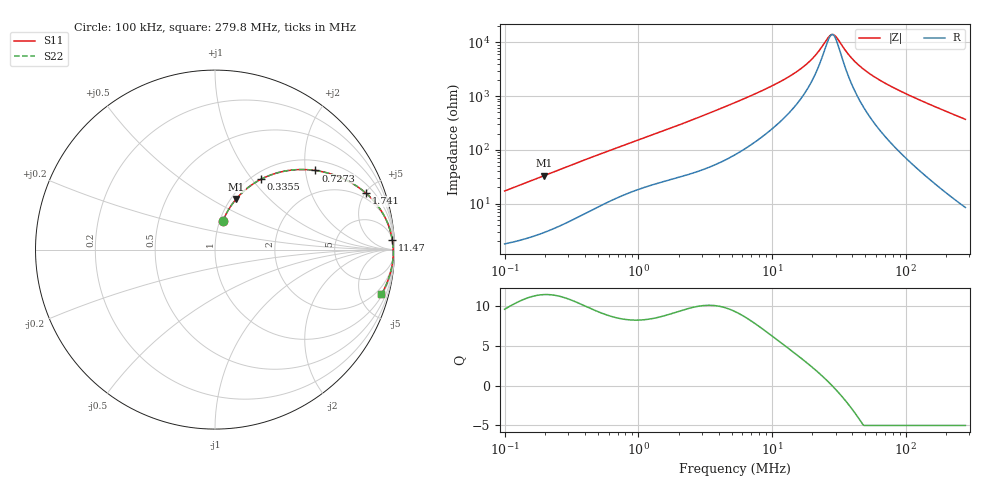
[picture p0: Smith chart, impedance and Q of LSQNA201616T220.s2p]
! LSQNA201616T220  S-PARAMETER MODEL  ( General Type )
! Model Generated by TAIYO YUDEN Corporation (http://www.ty-top.com)
! Version 2.0
! TAIYO YUDEN Control No. 100810NF25SB-FKC
! Copyright(c) 2007 TAIYO YUDEN CO.,LTD. All Rights Reserved.
! Product Description (link to TY-COMPAS)
! https://ds.yuden.co.jp/TYCOMPAS/or/detail?pn=LSQNA201616T220K&u=M
! Products Name : Inductors
! Characteristics :
!  Inductance : 22 uH , SRF(min) : 16 MHz , DC Resistance(max) : 1.3 Ohm
!  Rated Current : Saturation :165 mA , Temp Rise : 370 mA (40 degC)
!  Case Size : 2.0 x 1.6 / 0.079 x 0.063 [mm/inch] , Thickness : 1.6 / 0.063 [mm/inch]
!  (Conditions: Temperature = 25 degC , DC Bias Current/Voltage = 0A / 0V)
! External Node Assignments :
!  1  o---GGG---o  2
! GND o---------o GND
! Frequency Range : 0.1MHz  -  279.750408MHz  [ 402 STEP ]
# MHz S RI R 50
! Freq[MHz].  S11 Real  S11 Imag  S21 Real  S21 Imag  S12 Real  S12 Imag  S22 Real  S22 Imag
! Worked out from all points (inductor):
!   401 points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, 100 kHz to 279.8 MHz, reference 50 ohm
!   read as one part in series: L = 27 uH near 104 kHz
!   highest Q = 11.5 at 196.3 kHz (marker M1), where L = 26.8 uH
!   self-resonance near 28 MHz
!   S11 on the Smith chart (normalised r, x): 100 kHz: 1.04, +0.34; 335.5 kHz: 1.10, +1.11; 727.3 kHz: 1.27, +2.27; 1.741 MHz: 1.56, +5.04; 11.47 MHz: 8, +37; 279.8 MHz: 1.17, -7.42
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0.1  0.0444 0.1604  0.9556 -0.1604  0.9556 -0.1604  0.0444 0.1604
0.196325  0.1188 0.2828  0.8812 -0.2828  0.8812 -0.2828  0.1188 0.2828
0.335454  0.2559 0.3917  0.7441 -0.3917  0.7441 -0.3917  0.2559 0.3917
0.377863  0.2975 0.4108  0.7025 -0.4108  0.7025 -0.4108  0.2975 0.4108
0.727265  0.5598 0.4407  0.4402 -0.4407  0.4402 -0.4407  0.5598 0.4407
1.427803  0.7906 0.3529  0.2094 -0.3529  0.2094 -0.3529  0.7906 0.3529
1.741155  0.84 0.3154  0.16 -0.3154  0.16 -0.3154  0.84 0.3154
2.859306  0.924 0.2197  0.076 -0.2197  0.076 -0.2197  0.924 0.2197
5.289144  0.9701 0.1249  0.0299 -0.1249  0.0299 -0.1249  0.9701 0.1249
11.46689  0.9877 0.0519  0.0123 -0.0519  0.0123 -0.0519  0.9877 0.0519
15.7513  0.9904 0.0316  0.00956 -0.0316  0.00956 -0.0316  0.9904 0.0316
19.9857  0.9918 0.0182  0.00822 -0.0182  0.00822 -0.0182  0.9918 0.0182
22.51236  0.9923 0.0118  0.00771 -0.0118  0.00771 -0.0118  0.9923 0.0118
26.38496  0.9928 0.00347  0.0072 -0.00347  0.0072 -0.00347  0.9928 0.00347
28.56434  0.993 -0.000705  0.00701 0.000705  0.00701 0.000705  0.993 -0.000705
30.31621  0.9931 -0.00385  0.00689 0.00385  0.00689 0.00385  0.9931 -0.00385
36.96955  0.9933 -0.0146  0.00671 0.0146  0.00671 0.0146  0.9933 -0.0146
44.19738  0.9932 -0.0249  0.00685 0.0249  0.00685 0.0249  0.9932 -0.0249
56.07892  0.9924 -0.0399  0.00756 0.0399  0.00756 0.0399  0.9924 -0.0399
75.51853  0.9904 -0.062  0.00962 0.062  0.00962 0.062  0.9904 -0.062
136.9498  0.9786 -0.1241  0.0214 0.1241  0.0214 0.1241  0.9786 -0.1241
279.7504  0.9273 -0.2484  0.0727 0.2484  0.0727 0.2484  0.9273 -0.2484
